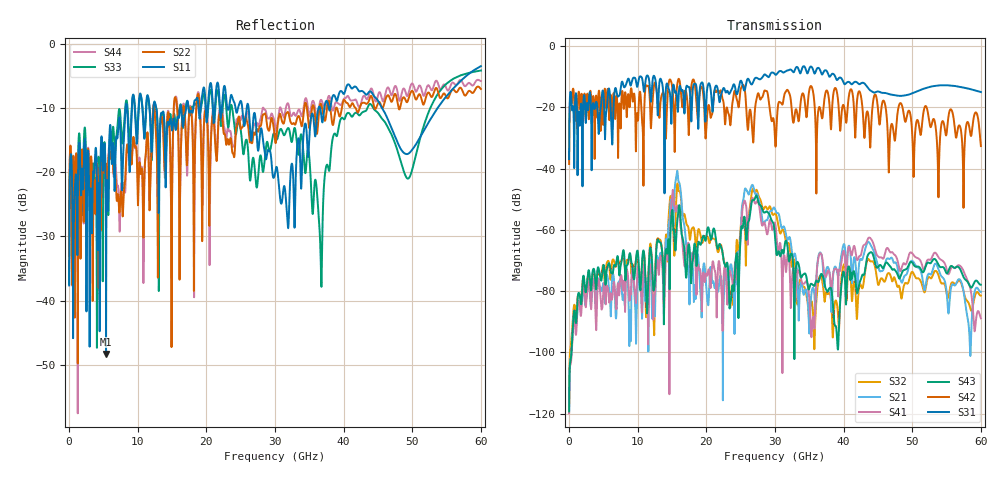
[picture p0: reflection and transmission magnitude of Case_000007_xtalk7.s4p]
! Info: Touchstone file created by circ.  Input file=CasetestDOE_NRZ_template_000007.circ
# Hz S RI R 50
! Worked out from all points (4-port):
!   6000 points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, 10 MHz to 60 GHz, reference 50 ohm
!   strongest paths, dB at 10 MHz, 15.01 GHz, 30.01 GHz, 45.01 GHz, 60 GHz:
!     S31: -36.9, -17.1, -9.2, -14.8, -15.0
!     S42: -38.5, -13.1, -30.5, -20.6, -32.6
!     S43: -119.2, -53.6, -62.2, -72.2, -77.9
!     S41: -119.9, -49.1, -57.8, -68.6, -88.9
!     S21: -119.2, -50.5, -53.2, -71.8, -80.2
!     S32: -116.9, -51.9, -54.6, -77.8, -81.5
!   lowest |S11| = -48.4 dB at 5.39 GHz (marker M1), VSWR 1.01, Z = 50.4 + j0.154 ohm
!   |S11| at or under -10 dB: start of sweep to 8.235 GHz; 26.17 GHz to 36.33 GHz (10.16 GHz wide, 32.5 % of centre); 45.61 GHz to 53.66 GHz (8.057 GHz wide, 16.2 % of centre)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
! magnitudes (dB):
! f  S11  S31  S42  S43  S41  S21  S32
! 10 MHz  -37.6  -36.9  -38.5  -119.2  -119.9  -119.2  -116.9
! 5.39 GHz  -48.4  -22.0  -19.6  -75.8  -81.6  -76.4  -72.7
! 15.78 GHz  -11.5  -19.3  -12.3  -57.0  -52.1  -40.8  -44.9
! 18.29 GHz  -8.8  -12.3  -12.1  -64.4  -67.8  -78.2  -60.7
! 23.83 GHz  -8.5  -13.3  -18.2  -78.1  -77.7  -75.0  -81.8
! 26.67 GHz  -14.2  -12.4  -26.6  -50.5  -49.7  -45.3  -47.1
! 60 GHz  -3.4  -15.0  -32.6  -77.9  -88.9  -80.2  -81.5
